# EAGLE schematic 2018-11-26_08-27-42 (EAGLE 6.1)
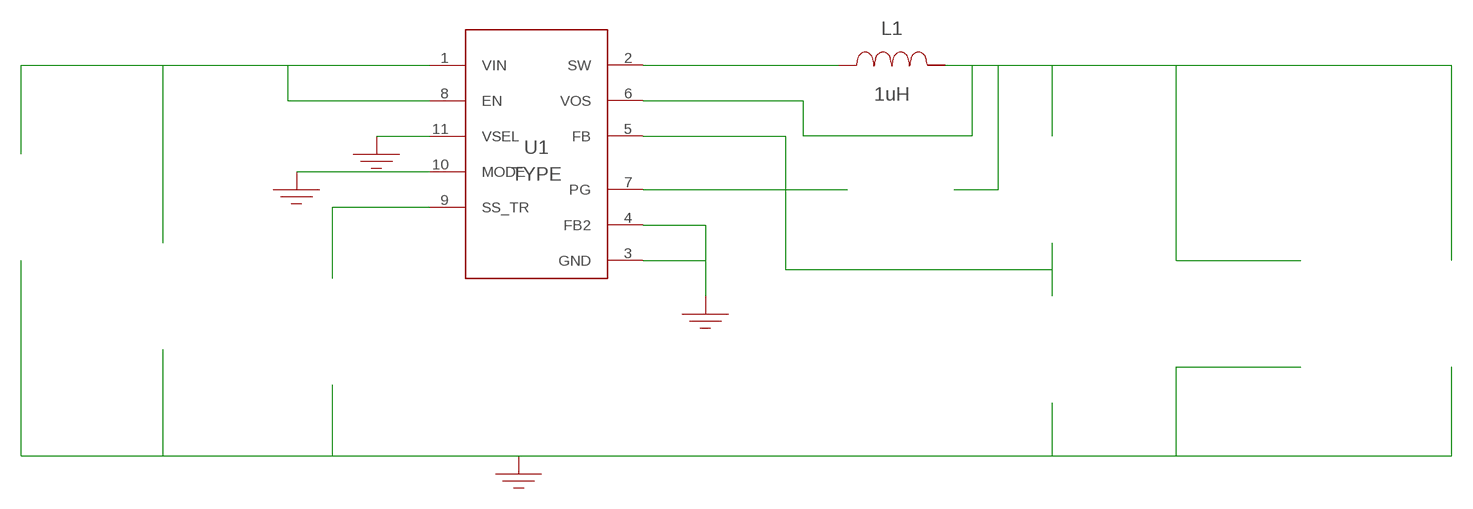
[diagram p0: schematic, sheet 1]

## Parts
CIN  6.8uF  C2012X5R1V685K125ACC2012X5R1V685K125AC  [0805]  (not placed on a sheet)
COUT  4.7uF  C2012X7R1V475K125ACC2012X7R1V475K125AC  [0805]  (not placed on a sheet)
COUT_2  4.7uF  C2012X7R1V475K125ACC2012X7R1V475K125AC  [0805]  (not placed on a sheet)
CSS  2.2nF  GRM155R61C222KA01DGRM155R61C222KA01D  [0402]  (not placed on a sheet)
GND  WB_GND  WB_GNDWB_GND  [WB_GND]
GND1  WB_GND  WB_GNDWB_GND  [WB_GND]
GND2  WB_GND  WB_GNDWB_GND  [WB_GND]
GND3  WB_GND  WB_GNDWB_GND  [WB_GND]
IOUT  WB_CURRENT_LOAD  WB_CURRENT_LOADWB_CURRENT_LOAD  [WB_CURRENT_LOAD]  (not placed on a sheet)
L1  1uH  XAL4020-102MEBXAL4020-102MEB  [XAL4020]
RFBB  100k  CRCW0402100KFKEDCRCW0402100KFKED  [0402]  (not placed on a sheet)
RFBT  1.62M  CRCW04021M62FKEDCRCW04021M62FKED  [0402]  (not placed on a sheet)
RPG  100k  CRCW0402100KFKEDCRCW0402100KFKED  [0402]  (not placed on a sheet)
U1  TPS62135RGXR  TPS62135RGXRTPS62135RGXR  [RGX0011A]
VIN  WB_BATTERY  WB_BATTERYWB_BATTERY  [WB_BATTERY]  (not placed on a sheet)

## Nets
0: Cin.2@2 Cout.2@2 Cout_2.2@2 Css.2@2 GND1.1 GND2.1 GND3.1 GND.1 Iout.-@2 Rfbb.2@2 U1.3(GND) U1.4(FB2) U1.10(MODE) U1.11(VSEL) Vin.-@2
1: Cout.1@1 Cout_2.1@1 Iout.+@1 L1.2 Rfbt.1@1 Rpg.1@1 U1.6(VOS)
2: Css.1@1 U1.9(SS_TR)
3: Rfbb.1@1 Rfbt.2@2 U1.5(FB)
4: Rpg.2@2 U1.7(PG)
5: Cin.1@1 U1.1(VIN) U1.8(EN) Vin.+@1
6: L1.1 U1.2(SW)
Unconnected: CIN.1 CIN.2 COUT.1 COUT.2 COUT_2.1 COUT_2.2 CSS.1 CSS.2 IOUT.1(+) IOUT.2(-) RFBB.1 RFBB.2 RFBT.1 RFBT.2 RPG.1 RPG.2 VIN.1(+) VIN.2(-)

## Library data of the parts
CIN = AcceleratedDesigns_Lib:C2012X5R1V685K125AC; Cap: 6.8E-6; Datasheet_URL: https://product.tdk.com/en/search/capacitor/ceramic/mlcc/info?part%5Fno%3DC2012X5R1V685K125AC; ESR: 0.003795; IRMS: 3.34931; Manufacturer_Name: TDK; Manufacturer_Part_Number: C2012X5R1V685K125AC; VDC: 35.0; Vendor: TDK
COUT COUT_2 = AcceleratedDesigns_Lib:C2012X7R1V475K125AC; Cap: 4.7E-6; Datasheet_URL: https://product.tdk.com/en/search/capacitor/ceramic/mlcc/info?part%5Fno%3DC2012X7R1V475K125AC; ESR: 0.002346; IRMS: 4.26021; Manufacturer_Name: TDK; Manufacturer_Part_Number: C2012X7R1V475K125AC; VDC: 35.0; Vendor: TDK
CSS = AcceleratedDesigns_Lib:GRM155R61C222KA01D; Cap: 2.2E-9; ESR: 0.0; IRMS: 0.0; Manufacturer_Name: MuRata; Manufacturer_Part_Number: GRM155R61C222KA01D; VDC: 16.0; Vendor: MuRata
GND GND1-GND3 = AcceleratedDesigns_Lib:WB_GND; Manufacturer_Name: WB_GND; Manufacturer_Part_Number: WB_GND; PowerPortType: POWER_GROUND; Value: Value
IOUT = AcceleratedDesigns_Lib:WB_CURRENT_LOAD; Manufacturer_Name: WB_CURRENT_LOAD; Manufacturer_Part_Number: WB_CURRENT_LOAD; PowerPortType: POWER_GROUND; Value: Value
L1 = AcceleratedDesigns_Lib:XAL4020-102MEB; DCR: 0.01; IDC: 8.75; L: 1.0E-6; Manufacturer_Name: Coilcraft; Manufacturer_Part_Number: XAL4020-102MEB; Vendor: Coilcraft
RFBB RPG = AcceleratedDesigns_Lib:CRCW0402100KFKED; Manufacturer_Name: Vishay-Dale; Manufacturer_Part_Number: CRCW0402100KFKED; Power: 0.063; Resistance: 100000.0; Tolerance: 1.0; Vendor: Vishay-Dale
RFBT = AcceleratedDesigns_Lib:CRCW04021M62FKED; Manufacturer_Name: Vishay-Dale; Manufacturer_Part_Number: CRCW04021M62FKED; Power: 0.063; Resistance: 1620000.0; Tolerance: 1.0; Vendor: Vishay-Dale
U1 = AcceleratedDesigns_Lib:TPS62135RGXR; Manufacturer: Texas Instruments; Manufacturer_Name: Texas Instruments; Manufacturer_Part_Number: TPS62135RGXR; PartNumber: TPS62135RGXR; RefDes: RefDes; TYPE: TYPE; Value: Value
VIN = AcceleratedDesigns_Lib:WB_BATTERY; Manufacturer_Name: WB_BATTERY; Manufacturer_Part_Number: WB_BATTERY; PowerPortType: POWER_GROUND; Value: Value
